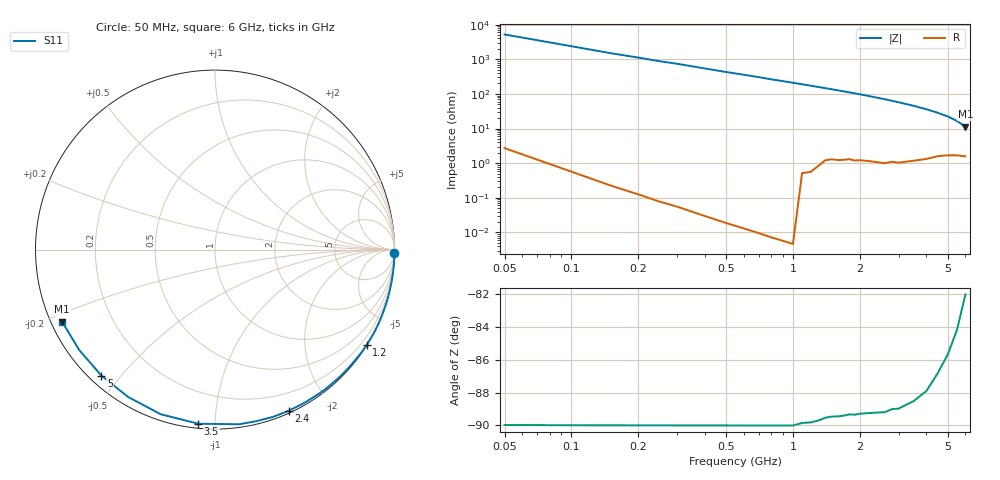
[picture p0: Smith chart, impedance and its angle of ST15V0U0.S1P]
! SIEMENS Discrete & RF Semiconductors
! BA892
! Si PIN Diode in SCD-80
! VR = 15 V
! S-Parameters:  September  1997
# GHz  S  MA  R  50
!  f  S11
! GHz  MAG  ANG
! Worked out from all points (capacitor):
!   34 points, 50 MHz to 6 GHz, reference 50 ohm
!   read as one part to ground: C = 667 fF near 50 MHz
!   lowest |Z| = 11.3 ohm at 6 GHz (marker M1)
!   S11 on the Smith chart (normalised r, x): 50 MHz: open; 1.2 GHz: 0.01, -3.46; 2.4 GHz: 0.02, -1.55; 3.5 GHz: 0.02, -0.91; 5 GHz: 0.03, -0.44; 6 GHz: 0.03, -0.22
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0.05  1 -1.1
0.2  1 -5.1
0.25  1 -6.5
0.3  1 -7.7
0.4  1 -10.5
0.5  1 -13.3
0.6  1 -15.9
0.7  1 -18.6
0.8  1 -21.5
1  1 -26.8
1.2  0.9983 -32.2
1.3  0.997 -35.0
1.5  0.9939 -40.3
1.6  0.9934 -43.2
1.8  0.9911 -48.7
1.9  0.9911 -51.4
2  0.9899 -54.2
2.2  0.9886 -59.8
2.4  0.9875 -65.5
2.6  0.9867 -71.0
2.8  0.9832 -76.7
3  0.9823 -82.2
3.5  0.9745 -95.5
4  0.9657 -108.3
4.5  0.9531 -120.5
5  0.9452 -132.0
5.5  0.941 -143.5
6  0.942 -154.8
